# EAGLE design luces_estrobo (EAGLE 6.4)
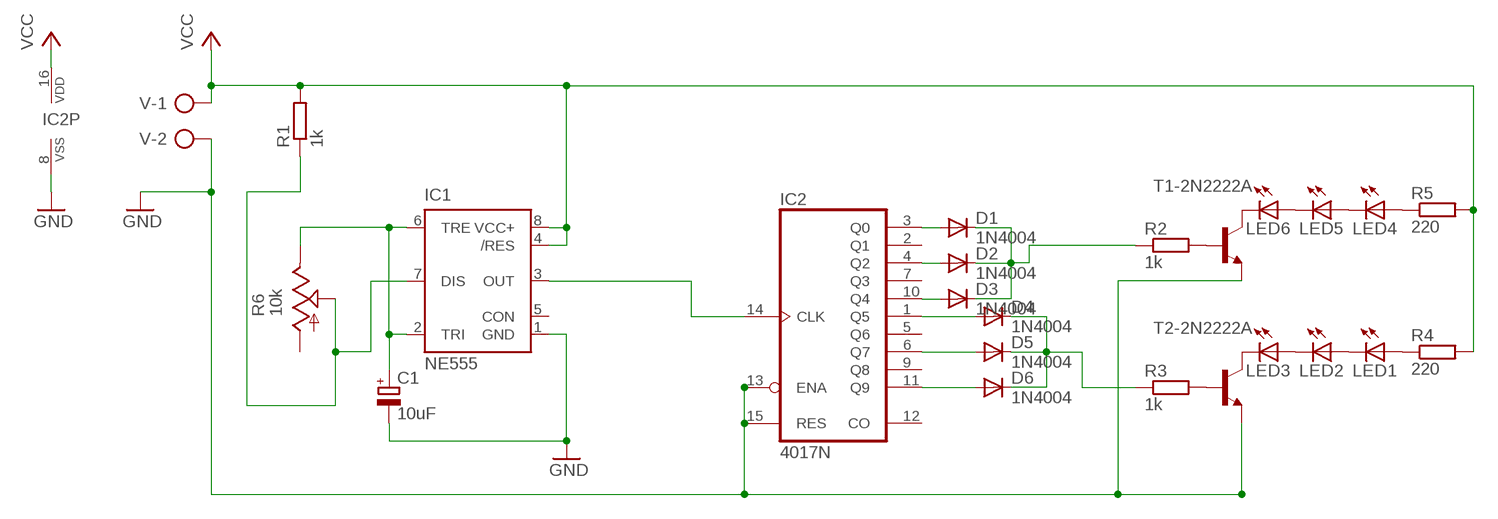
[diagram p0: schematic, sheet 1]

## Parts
C1  10uF  CPOL-EUE2.5-6  [E2,5-6]
D1  1N4004  [DO41-10]
D2  1N4004  [DO41-10]
D3  1N4004  [DO41-10]
D4  1N4004  [DO41-10]
D5  1N4004  [DO41-10]
D6  1N4004  [DO41-10]
IC1  NE555  [DIL-08]
IC2  4017N  [DIL16]
LED1  LED5MM  [LED5MM]
LED2  LED5MM  [LED5MM]
LED3  LED5MM  [LED5MM]
LED4  LED5MM  [LED5MM]
LED5  LED5MM  [LED5MM]
LED6  LED5MM  [LED5MM]
R1  1k  R-EU_0207/10  [0207/10]
R2  1k  R-EU_0207/10  [0207/10]
R3  1k  R-EU_0207/10  [0207/10]
R4  220  R-EU_0207/10  [0207/10]
R5  220  R-EU_0207/10  [0207/10]
R6  10k  TRIM_US-CA6V  [CA6V]
T1-2N2222A  -NPN-TO92-EBC  [TO92-EBC]
T2-2N2222A  -NPN-TO92-EBC  [TO92-EBC]
V  AK500/2  [AK500/2]

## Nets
GND: C1.- IC1.1(GND) IC2.8(VSS) IC2.13(ENA) IC2.15(RES) T1-2N2222A.E T2-2N2222A.E V.2
N$1: D1.A IC2.3(Q0)
N$2: D2.A IC2.4(Q2)
N$3: D3.A IC2.10(Q4)
N$4: D4.A IC2.1(Q5)
N$5: D5.A IC2.6(Q7)
N$6: D6.A IC2.11(Q9)
N$7: LED1.K(C) LED2.A
N$8: LED2.K(C) LED3.A
N$9: LED4.K(C) LED5.A
N$10: LED5.K(C) LED6.A
N$11: R2.2 T1-2N2222A.B
N$12: R3.2 T2-2N2222A.B
N$13: D1.C D2.C D3.C R2.1
N$14: LED1.A R4.1
N$15: D4.C D5.C D6.C R3.1
N$16: LED4.A R5.1
N$17: LED6.K(C) T1-2N2222A.C
N$18: LED3.K(C) T2-2N2222A.C
N$19: IC1.3(OUT) IC2.14(CLK)
N$20: C1.+ IC1.2(TRI) IC1.6(TRE) R6.E
N$22: IC1.7(DIS) R1.1 R6.S
VCC: IC1.4(/RES) IC1.8(VCC+) IC2.16(VDD) R1.2 R4.2 R5.2 V.1
Unconnected: IC1.5(CON) IC2.2(Q1) IC2.5(Q6) IC2.7(Q3) IC2.9(Q8) IC2.12(CO) R6.A

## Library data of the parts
C1 = rcl:CPOL-EU: POLARIZED CAPACITOR, European symbol
D1-D6 = diode:1N4004: DIODE
IC1 = st-microelectronics:NE555: General purpose bipolar Timer; MF: Arrow Electronics; MPN: NE555N; OC_FARNELL: 1467742; OC_NEWARK: 89K1486
IC2 = 40xx:4017: COUNTER/DIVIDER
LED1-LED6 = led:LED: LED
R1-R5 = rcl:R-EU_: RESISTOR, European symbol
R6 = pot:TRIM_US-: POTENTIOMETER
T1-2N2222A T2-2N2222A = transistor:*-NPN-: NPN Transistror BF959 corrected 2008.03.06
V = con-ptr500:AK500/2: CONNECTOR; OC_FARNELL: unknown; OC_NEWARK: unknown

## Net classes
0 default: clearance 0.355 mm

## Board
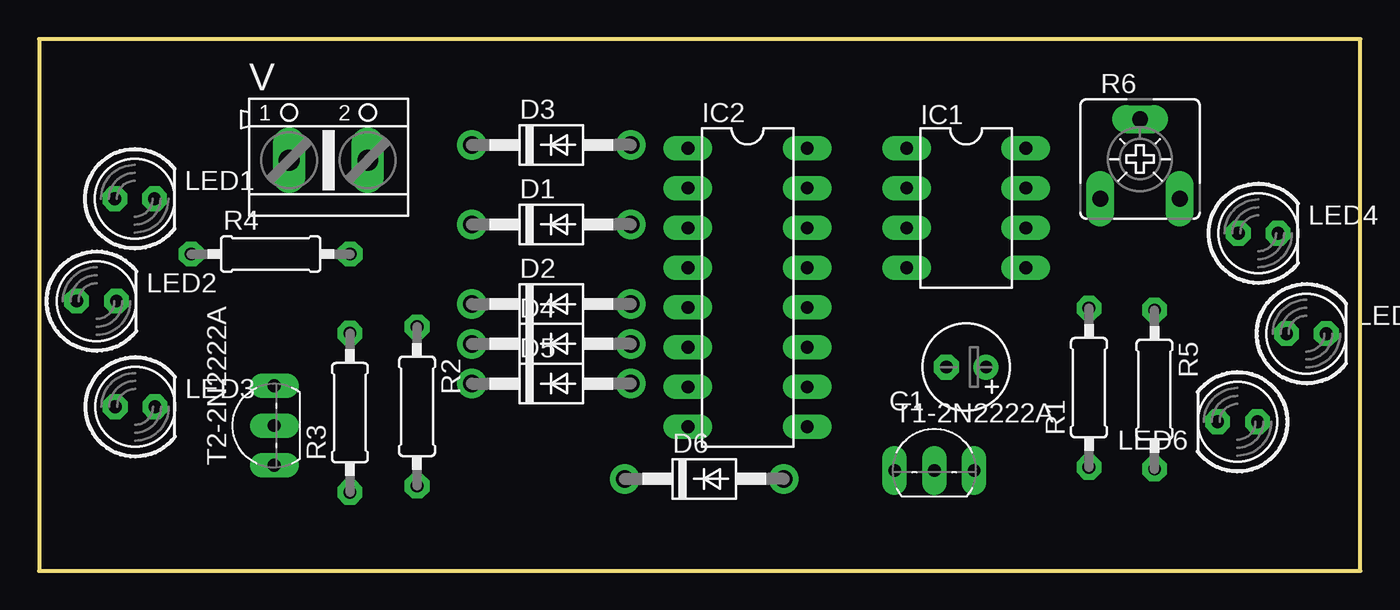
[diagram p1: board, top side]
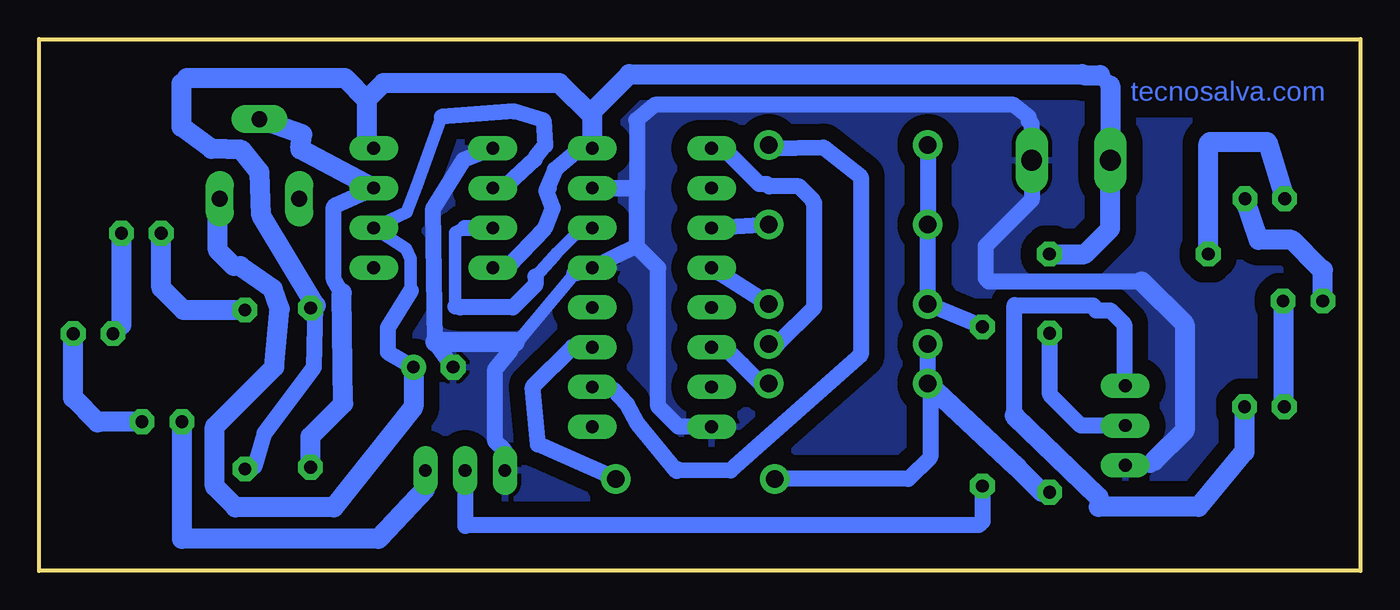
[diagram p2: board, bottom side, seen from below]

Size 84.43 x 33.96 mm. Coordinates in mm from the lower left corner, seen from the top.
Outline: 0,0 84.42,0 84.43,33.96 0,33.96 0,0
Copper layers (1*16): Top 0.035mm / dielectric 1.5mm / Bottom 0.035mm
Design rules "default": minimum track width 22mil, minimum drill 24mil, track to track 8mil, track to pad 8mil, pad to pad 8mil, via to via 8mil, smd to smd 8mil, copper to edge 40mil, drill to drill 8mil, minimum pad ring 15mil, minimum via ring 8mil, stop-mask expansion 4mil, vias tented up to drill 0mil, thermal gap 10mil

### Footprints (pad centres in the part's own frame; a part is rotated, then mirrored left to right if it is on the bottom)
E2,5-6 = drill 0.813 pad 1.6: + -1.27,0 | drill 0.813 pad 1.6 octagon: - 1.27,0
DO41-10 = drill 1.118: A 5.08,0; C -5.08,0
DIL-08 = drill 0.813 long: 1 -3.81,-3.81; 2 -1.27,-3.81; 3 1.27,-3.81; 4 3.81,-3.81; 5 3.81,3.81; 6 1.27,3.81; 7 -1.27,3.81; 8 -3.81,3.81
DIL16 = drill 0.813 long: 1 -8.89,-3.81; 2 -6.35,-3.81; 3 -3.81,-3.81; 4 -1.27,-3.81; 5 1.27,-3.81; 6 3.81,-3.81; 7 6.35,-3.81; 8 8.89,-3.81; 9 8.89,3.81; 10 6.35,3.81; 11 3.81,3.81; 12 1.27,3.81; 13 -1.27,3.81; 14 -3.81,3.81; 15 -6.35,3.81; 16 -8.89,3.81
LED5MM = drill 0.813 octagon: A -1.27,0; K 1.27,0
0207/10 = drill 0.813 octagon: 1 -5.08,0; 2 5.08,0
CA6V = drill 1.016 long: A -2.54,-2.54; E 2.54,-2.54; S 0,2.54
TO92-EBC = drill 0.813 long: B 0,-1.27; C 2.54,-1.27; E -2.54,-1.27
AK500/2 = drill 1.321 long: 1 -2.515,0; 2 2.515,0

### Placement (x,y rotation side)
C1  59.24,13.01 180 top
D1  32.72,22.12 0 top
D2  32.72,17.04 0 top
D3  32.72,27.2 0 top
D4  32.72,14.5 0 top
D5  32.72,11.96 0 top
D6  42.5,5.87 0 top
IC1  59.24,23.17 270 top
IC2  45.27,18.09 270 top
LED1  6.11,23.77 0 top
LED2  3.67,17.23 0 top
LED3  6.13,10.47 0 top
LED4  77.9,21.56 0 top
LED5  80.98,15.15 0 top
LED6  76.58,9.52 180 top
R1  67.08,11.7 90 top
R2  24.15,10.5 270 top
R3  19.86,10.1 90 top
R4  14.8,20.24 0 top
R5  71.27,11.58 270 top
R6  70.35,26.3 0 top
T1-2N2222A  57.2,7.68 0 top
T2-2N2222A  13.75,9.28 90 top
V  18.49,26.23 0 top

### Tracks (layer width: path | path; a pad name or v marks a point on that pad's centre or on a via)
GND
  Bottom 0.559: 14.79,6.66 T2-2N2222A.E | 54.04,14.61 54.15,14.28
  Bottom 0.813: 54.27,14.12 54.15,14.28 50.22,18.98
  Bottom 1.016: 46.26,20.73 46.26,24.44 IC2.15 46.21,24.44 46.21,28.78 46.26,28.78 45.09,29.76 22.15,29.76 21.19,28.99 21.19,28.74 21,28.55 V.2 21,23.69 23.95,20.74 23.95,18.69 23.75,18.49 13.98,18.49 | 46.26,20.73 IC2.13 50.22,18.98 | IC2.8 43.58,9.2 44.88,10.5 44.88,19.35 46.26,20.73 | 13.18,7.02 | 13.18,7.02 13.43,6.77 14.99,6.77 T2-2N2222A.E | T1-2N2222A.E 54.66,7.65 55.28,8.27 55.28,12.88 54.27,14.12 | C1.- 59.12,14.61 59.24,23.17 57.32,26.24 IC1.1
  Bottom 1.27: 13.98,18.49 11.23,15.74 11.23,8.98 13.18,7.02 | 54.04,14.61 59.12,14.61
  pour Bottom (isolate 1.016): 0.06,33.92 0.01,33.92 0.01,-0.21
  pour Bottom (isolate 1.016): 0.06,33.92 0.06,0.04 84.57,0.04 84.57,0.15 84.37,0.15 84.37,34.02 0.11,34.02 0.11,33.72
N$1
  Bottom 0.559: 37.65,21.9 D1.A
  Bottom 1.016: IC2.3 D1.A
N$2
  Bottom 1.016: D2.A IC2.4
N$3
  Bottom 0.559: 37.65,26.98 D3.A | IC2.10 49.08,11.57
  Bottom 1.016: 37.65,26.98 34.32,27.04 31.92,25.16 31.92,13.8 40.24,6.42 43.58,6.4 43.59,6.46 43.7,6.36 46.18,9.39 46.85,10.63 47.72,11.57 49.08,11.57 49.09,11.57 | 47.87,11.58 48.91,11.58 IC2.10
N$4
  Bottom 1.016: D4.A 37.23,14.5 34.89,16.84 34.89,23.48 35,23.58 35,23.69 35.87,24.56 37.78,24.56 37.92,24.7 38.4,24.7 40.52,26.82 41.29,26.82 IC2.1
N$5
  Bottom 1.016: D5.A 38.29,11.96 39.5,13.17 | 39.5,13.17 | 39.5,13.17 40.46,14.13 41.31,14.13 IC2.6
N$6
  Bottom 1.016: D6.A 52.55,8.08 52.89,11.74 50.35,14.28 IC2.11
N$7
  Bottom 1.016: 2.4,19.21 2.53,19.34 2.58,19.34
  Bottom 1.27: LED2.A 2.4,19.21 | 2.58,19.34 4.39,21.14 6.49,21.14 LED1.K
N$8
  Bottom 1.016: 4.94,10.55 LED3.A
  Bottom 1.27: LED2.K 4.94,10.55
N$9
  Bottom 1.27: LED4.K 79.17,15.69 LED5.A
N$10
  Bottom 1.016: 80.54,9.52 80.58,9.48 80.7,9.48 | 82.26,15.14 LED5.K
  Bottom 1.27: LED6.A 80.54,9.52 | 80.7,9.48 82.26,11.04 82.26,15.14
N$11
  Bottom 1.016: R2.2 24.15,3.41 24.14,3.4 24.14,3.16 24.38,2.92 57.12,2.92 57.18,2.86 57.18,6.39 T1-2N2222A.B
N$12
  Bottom 1.016: T2-2N2222A.B 17.86,9.28 19.83,11.25 19.83,15.15 R3.2
N$13
  Bottom 1.016: D3.C D1.C D2.C R2.1
N$14
  Bottom 1.016: 9.72,27.29 9.62,27.39
  Bottom 1.27: R4.1 9.72,27.29 | 9.62,27.39 5.95,27.39 LED1.A
N$15
  Bottom 0.559: 27.49,11.74 D5.C | 27.49,13.01 27.64,13.01
  Bottom 1.016: D5.C 27.64,13.01 D4.C | 27.49,11.74 27.49,7.27 28.89,5.87 D6.C | R3.1 20.34,5.02
  Bottom 1.27: 20.34,5.02 21.94,6.62 D5.C
N$16
  Bottom 1.016: 76.61,21.54 LED4.A
  Bottom 1.27: R5.1 75.2,16.66 76.61,18.07 76.61,21.54
N$17
  Bottom 1.016: T1-2N2222A.C 59.74,5.25 | 75.3,2.04 75.29,2.26 | 75.29,9.5 LED6.K
  Bottom 1.27: 59.74,5.25 62.74,2.04 75.3,2.04 | 75.29,2.26 75.29,9.5
N$18
  Bottom 0.559: 16.06,11.74 T2-2N2222A.C
  Bottom 1.016: 16.74,4.09 16.74,4.72 | 22.11,9.92 22.11,16.98 21.49,16.95 17.09,16.95 16.89,16.64 15.99,16.64 15.08,15.74 15.08,11.88 T2-2N2222A.C
  Bottom 1.27: LED3.K 7.4,7.59 10.33,4.09 16.74,4.09 | 16.74,4.72 22.11,9.92
N$19
  Bottom 0.813: 57.84,16.87 57.84,21.59 57.24,21.91 | 49.74,21.9 51.37,20.28 51.49,20.14 52.72,18.79
  Bottom 1.016: 57.84,16.87 57.51,16.82 54.16,16.82 52.72,18.26 52.72,18.79 | 57.24,21.91 IC1.3 | IC2.14 49.74,21.9
N$20
  Bottom 0.813: 58.7,28.99 60.31,24.58 60.94,22.91 IC1.6 60.98,20.56 60.69,19.93 60.69,17.89
  Bottom 1.016: 58.7,28.99 54.07,29.35 52.2,28.78 52.08,27.18 52.73,26.38 52.76,26.28 54.93,24.28 55.26,24.28 IC1.2 | 71.57,19.46 71.99,19.46 | 73.01,23.64 R6.E | 60.69,17.89 62.15,15.51 62.15,13.97 C1.+
  Bottom 1.27: C1.+ 60.51,10.47 65.61,4.05 71.87,4.05 73.21,5.39 73.21,9.2 69.4,13.01 69.05,16.72 69.49,18.01 71.57,19.46 | 71.99,19.46 73.01,20.48 73.01,23.64
N$22
  Bottom 1.016: 65.09,17.74 65.6,18.62 65.6,23.24 65.48,23.36 IC1.7
  Bottom 1.27: R1.1 67.08,8.59 65,10.68 65.09,17.74 | IC1.7 67.74,26.91 67.62,27.88 R6.S
VCC
  Bottom 0.559: 15.98,25.71 16.06,25.71 V.1 | 66.74,16.94 R1.2
  Bottom 1.016: 51.85,24.44 52.02,24.28 | 52.02,24.28 51.62,23.17 52.13,21.86 54.5,19.4 IC1.4 | 52.02,24.28 51.47,25.62 49.84,26.98 IC2.16 49.08,29.06 | 15.98,25.71 V.1 | R5.2 70.67,6.66 70.04,8.77 66.86,13.01 66.74,16.94 | 75.33,31.12 74.97,31.48 | 63.5,27.43 IC1.8 | 17.79,31.73 17.72,31.66 | 16.63,31.66 15.99,31.01 | 15.99,26.24 V.1
  Bottom 1.27: R4.2 17.61,20.24 15.98,21.86 15.98,25.71 | 66.74,16.94 70.23,22.7 70.34,25.47 71.49,26.89 73.41,26.96 75.33,28.35 75.33,31.12 | 74.97,31.48 64.88,31.48 63.5,30.1 | 63.5,30.1 63.5,27.43 | 49.08,29.06 51.17,31.16 62.44,31.16 63.5,30.1 | IC2.16 49.08,29.36 46.7,31.73 17.79,31.73 | 17.72,31.66 16.63,31.66 | 15.99,31.01 15.99,26.24

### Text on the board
Bottom: tecnosalva.com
